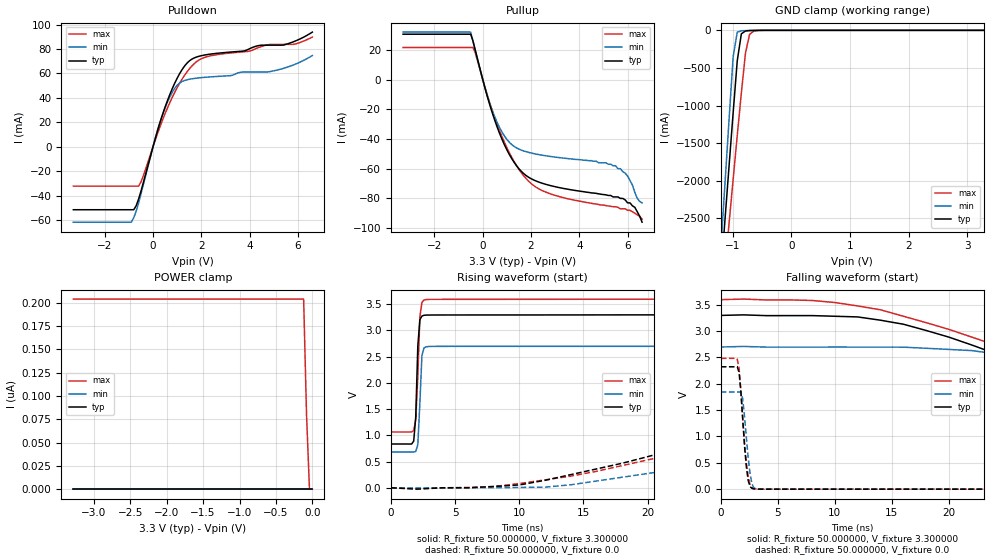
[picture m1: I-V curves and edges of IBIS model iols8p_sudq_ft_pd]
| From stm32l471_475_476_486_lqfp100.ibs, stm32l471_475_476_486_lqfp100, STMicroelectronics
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|   Model iols8p_sudq_ft_pd
[Model]  iols8p_sudq_ft_pd
Model_type I/O
Polarity   Non-Inverting
Enable   Active-Low
Vinl =   0.990000V
Vinh =   2.310000V
Vmeas =  1.650000V
Cref =   50.000000pF
Rref =   100.000000M
Vref =   0.0V
C_comp   2.036400pF   1.984000pF   2.082300pF
[Temperature Range]   25.000000   -40.000000   0.125000k
[Pullup Reference]   3.300000V   2.700000V   3.600000V
[Pulldown Reference]   0.0V   0.0V   0.0V
[POWER Clamp Reference]   3.300000V   2.700000V   3.600000V
[GND Clamp Reference]   0.0V   0.0V   0.0V
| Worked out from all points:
|   slope of the pulldown table from 0 to 0.495 V, typ, clamps not added: 15.4 ohm
|   slope of the pullup table from 0 to 0.495 V, typ, clamps not added: 18.1 ohm
|   GND clamp passes 1 mA (typ) near -0.60 V on its own axis
|   rising waveform, R_fixture 50.000000, V_fixture 3.300000: 20-80 % time 204ps typ, 227ps min, 243ps max; typ from 0.835 V to 3.3 V
|   rising waveform, R_fixture 50.000000, V_fixture 0.0: 20-80 % time 24.4ns typ, 26.2ns min, 30.7ns max; typ from 0 V to 2.32 V
|   falling waveform, R_fixture 50.000000, V_fixture 3.300000: 20-80 % time 21.2ns typ, 25.4ns min, 24ns max; typ from 3.3 V to 0.835 V
|   falling waveform, R_fixture 50.000000, V_fixture 0.0: 20-80 % time 469ps typ, 493ps min, 522ps max; typ from 2.32 V to 0 V
[Pulldown]
|Voltage   I(typ)   I(min)   I(max)
-3.3V     -51.62mA   -61.83mA   -32.32mA
-900mV    -51.62mA   -61.83mA   -32.32mA
-800mV    -51.62mA   -58.24mA   -32.32mA
-500mV    -36.51mA   -38.71mA   -28.96mA
400mV     26.66mA    26.58mA    22.18mA
800mV     47.72mA    44.74mA    40.6mA
1.1V      59.79mA    52.18mA    51.93mA
1.5V      70.22mA    55.24mA    63.66mA
2.1V      74.97mA    56.75mA    72.88mA
4.9V      83.19mA    61.75mA    83.83mA
5.9V      86.64mA    67.67mA    84.15mA
6.6V      93.9mA     74.68mA    89.84mA
[Pullup]
|Voltage   I(typ)   I(min)   I(max)
-3.3V     30.51mA    31.92mA    21.54mA
-500mV    30.51mA    31.92mA    21.54mA
-300mV    19.24mA    18.93mA    17.46mA
500mV     -27.53mA   -25.31mA   -25.83mA
1V        -47.29mA   -40.29mA   -45.86mA
1.5V      -60.05mA   -46.83mA   -60.43mA
2V        -66.7mA    -49.43mA   -69.91mA
2.7V      -70.92mA   -51.53mA   -76.32mA
5.5V      -79mA      -58mA      -85.6mA
6V        -83mA      -65mA      -88mA
6.3V      -86mA      -76mA      -90mA
6.6V      -96mA      -83mA      -94mA
[GND_clamp]
|Voltage   I(typ)   I(min)   I(max)
-3.3V     -9.812A    -9.822A    -9.937A
-1.2V     -3.251A    -2.905A    -3.763A
-1.13V    -2.527A    -2.046A    -3.165A
-1.06V    -1.808A    -1.191A    -2.57A
-990mV    -1.097A    -352.7mA   -1.979A
-920mV    -404.2mA   -25.09mA   -1.398A
-850mV    -46.54mA   -6.516mA   -832.3mA
-780mV    -8.509mA   -3.59mA    -302.4mA
-710mV    -3.395mA   -1.728mA   -53.82mA
-640mV    -1.602mA   -565.6uA   -11.73mA
-360mV    -11.48uA   -7.86uA    -95.15uA
3.28V     87.11uA    57.76uA    110.6uA
[POWER_clamp]
|Voltage   I(typ)   I(min)   I(max)
-3.28V    0A         0A         204.1nA
-120mV    0A         0A         204.1nA
-80mV     0A         0A         79.47nA
-40mV     0A         0A         0A
0V        0A         0A         0A
[Ramp]
| variable   typ   min   max
dV/dt_r  1.39392/24.32512n   1.10664/26.02554n   1.48968/30.68457n
dV/dt_f  1.47853/21.12242n   1.20971/25.31352n   1.52064/23.80312n
R_load = 50.000000
[Rising Waveform]
R_fixture= 50.000000
V_fixture= 3.300000
V_fixture_min= 2.700000
V_fixture_max= 3.600000
|time   V(typ)   V(min)   V(max)
0s        834.7mV    683mV      1.064V
1.602ns   834.4mV    682.6mV    1.065V
1.762ns   890.2mV    681.2mV    1.091V
1.922ns   1.358V     691.7mV    1.293V
2.082ns   2.701V     821.7mV    2.121V
2.242ns   3.204V     1.613V     3.263V
2.402ns   3.274V     2.525V     3.537V
2.563ns   3.289V     2.664V     3.579V
2.723ns   3.292V     2.686V     3.588V
79.76ns   3.299V     2.699V     3.598V
[Rising Waveform]
R_fixture= 50.000000
V_fixture= 0.0
V_fixture_min= 0.0
V_fixture_max= 0.0
|time   V(typ)   V(min)   V(max)
0s        2.52nV     1.819nV    187.9nV
10.01ns   54.08mV    6.364mV    80.09mV
14.01ns   251mV      56.77mV    221.9mV
22.02ns   729.2mV    344.7mV    640.7mV
34.03ns   1.484V     929.4mV    1.304V
46.05ns   1.975V     1.399V     1.852V
54.05ns   2.117V     1.595V     2.09V
62.06ns   2.197V     1.7V       2.223V
100.1ns   2.301V     1.827V     2.435V
997ns     2.323V     1.844V     2.483V
[Falling Waveform]
R_fixture= 50.000000
V_fixture= 3.300000
V_fixture_min= 2.700000
V_fixture_max= 3.600000
|time   V(typ)   V(min)   V(max)
0s        3.299V     2.699V     3.598V
10.01ns   3.283V     2.698V     3.543V
16.02ns   3.132V     2.696V     3.283V
24.02ns   2.579V     2.572V     2.74V
38.04ns   1.559V     1.933V     1.812V
46.05ns   1.181V     1.508V     1.457V
60.06ns   976.5mV    964.6mV    1.241V
82.08ns   892.5mV    775.2mV    1.135V
220.2ns   834.9mV    682.5mV    1.065V
997ns     834.7mV    683mV      1.064V
[Falling Waveform]
R_fixture= 50.000000
V_fixture= 0.0
V_fixture_min= 0.0
V_fixture_max= 0.0
|time   V(typ)   V(min)   V(max)
0s        2.323V     1.844V     2.483V
1.441ns   2.327V     1.844V     2.469V
1.602ns   2.214V     1.847V     2.292V
1.762ns   1.842V     1.846V     1.876V
1.922ns   1.323V     1.714V     1.35V
2.242ns   418.5mV    976.9mV    495.4mV
2.402ns   163.5mV    592.8mV    240.7mV
2.723ns   16.02mV    107.4mV    30.17mV
3.043ns   2.769mV    10.45mV    4.778mV
79.76ns   2.52nV     1.819nV    187.9nV
